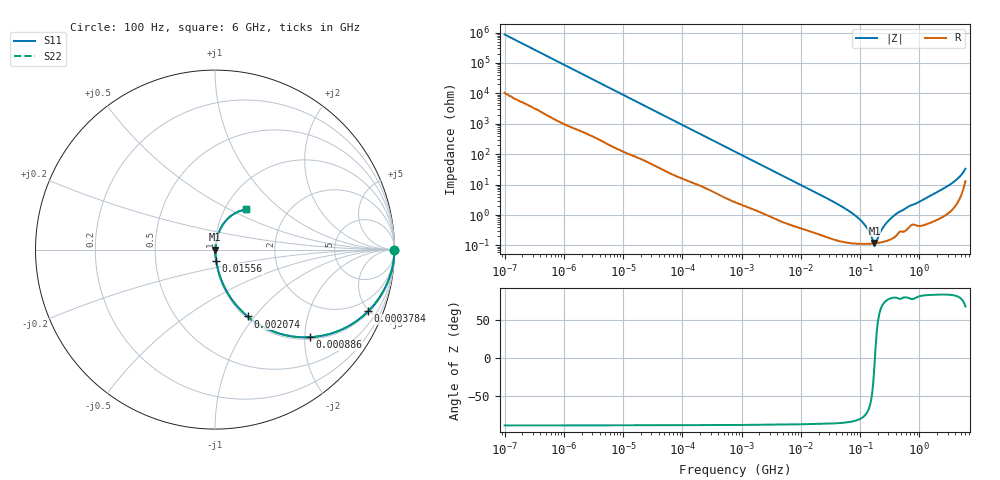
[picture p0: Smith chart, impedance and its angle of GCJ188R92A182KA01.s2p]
!Murata Part Number: GCJ188R92A182KA01
!These Parameters are Measured in Series Mode Connection
!Data Generated on Mar 13, 2026
!  o--ll--o
!Port1  Port2
!  o------o
!Operation Temp=25[degC], DC Bias Voltage=0[V]
!Freq. Start=100[Hz] Stop=6[GHz] 401[Steps]
# Hz S RI R 50
!Freq.(Hz) S11(Real) S11(Imag) S21(Real) S21(Imag) S12(Real) S12(Imag) S22(Real) S22(Imag)
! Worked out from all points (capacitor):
!   401 points, 100 Hz to 6 GHz, reference 50 ohm
!   read as one part in series: C = 1.83 nF near 109 Hz
!   lowest |Z| = 119 mohm at 174.6 MHz (marker M1)
!   series resonance near 178.3 MHz, so ESL is about 440 pH
!   S11 on the Smith chart (normalised r, x): 100 Hz: open; 378.4 kHz: 1.10, -4.93; 886 kHz: 1.05, -2.13; 2.074 MHz: 1.02, -0.92; 15.56 MHz: 1.01, -0.13; 6 GHz: 1.26, +0.61
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100  1 -0.000115  1.4e-06 0.000115  1.4e-06 0.000115  1 -0.000115
2008  1 -0.00227  3.37e-05 0.00227  3.37e-05 0.00227  1 -0.00227
40335  0.9973 -0.0442  0.00266 0.0442  0.00266 0.0442  0.9973 -0.0442
135116  0.9764 -0.143  0.0236 0.143  0.0236 0.143  0.9764 -0.143
378399  0.8538 -0.3432  0.1462 0.3432  0.1462 0.3432  0.8538 -0.3432
774597  0.5942 -0.4803  0.4058 0.4803  0.4058 0.4803  0.5942 -0.4803
885955  0.5303 -0.4881  0.4697 0.4881  0.4697 0.4881  0.5303 -0.4881
2074311  0.1813 -0.3722  0.8187 0.3722  0.8187 0.3722  0.1813 -0.3722
4440638  0.0507 -0.2052  0.9493 0.2052  0.9493 0.2052  0.0507 -0.2052
1.555665e7  0.00667 -0.0625  0.9933 0.0625  0.9933 0.0625  0.00667 -0.0625
4.556224e7  0.0018 -0.0206  0.9982 0.0206  0.9982 0.0206  0.0018 -0.0206
8.527865e7  0.00122 -0.00914  0.9988 0.00914  0.9988 0.00914  0.00122 -0.00914
1.220122e8  0.00114 -0.00441  0.9989 0.00441  0.9989 0.00441  0.00114 -0.00441
1.745687e8  0.00117 -0.000239  0.9988 0.000239  0.9988 0.000239  0.00117 -0.000239
1.909225e8  0.00119 0.00078  0.9988 -0.00078  0.9988 -0.00078  0.00119 0.00078
2.388273e8  0.0013 0.00338  0.9987 -0.00338  0.9987 -0.00338  0.0013 0.00338
3.124326e8  0.00155 0.00675  0.9984 -0.00675  0.9984 -0.00675  0.00155 0.00675
4.087225e8  0.00221 0.0107  0.9978 -0.0107  0.9978 -0.0107  0.00221 0.0107
6.395615e8  0.00385 0.018  0.9961 -0.018  0.9961 -0.018  0.00385 0.018
3.065283e9  0.0191 0.0881  0.9809 -0.0881  0.9809 -0.0881  0.0191 0.0881
4.586474e9  0.0522 0.1512  0.9478 -0.1512  0.9478 -0.1512  0.0522 0.1512
6e9  0.1748 0.2244  0.8252 -0.2244  0.8252 -0.2244  0.1748 0.2244
